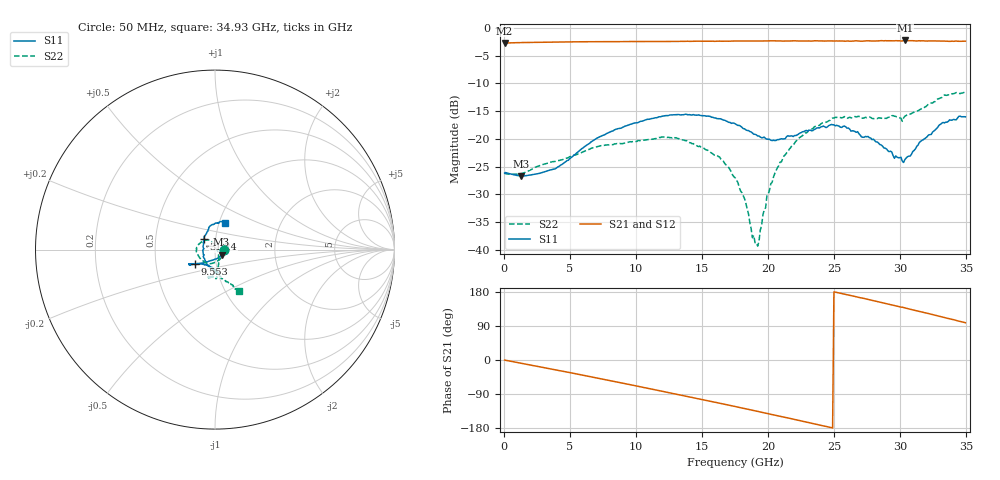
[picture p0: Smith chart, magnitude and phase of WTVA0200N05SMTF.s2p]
! 50 ohm 2-Port S-parameters measured by Modelithics Inc support@modelithics.com  Tampa, FL USA 813-866-6335 (February 2024)
! Smiths Interconnect,  2dB P/N: WTVA0200N05SMTF, Temperature: -25 C
! Board: 10 mil Rogers 4350B, Mounting Pad Dimensions: Length: 15 mils, Width: 25 mils, Gap: 40 mils.
# Hz S RI R 50
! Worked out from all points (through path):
!   352 points, 50 MHz to 34.93 GHz, reference 50 ohm
!   highest |S21| = -2.26 dB at 30.35 GHz (marker M1); lowest = -2.7 dB at 50 MHz (marker M2)
!   group delay of S21, straight-line fit = 20.8 ps
!   lowest |S11| = -26.7 dB at 1.294 GHz (marker M3), VSWR 1.10, Z = 53.7 - j3.05 ohm
!   |S11| at or under -10 dB: start of sweep to end of sweep
!   |S22| runs from -39.3 to -11.5 dB; largest |S21 - S12| = 0.0085
!   S11 on the Smith chart (normalised r, x): 50 MHz: 1.10, -0.00; 9.553 GHz: 0.79, -0.13; 31.24 GHz: 0.88, +0.11; 34.93 GHz: 1.07, +0.32
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5e7  0.0492 -0.00113  0.7303 -0.00271  0.7295 -0.00321  0.0499 -0.00106
1.2945e9  0.0368 -0.0283  0.7298 -0.1057  0.729 -0.1059  0.0395 -0.0285
3.8815e9  -0.00116 -0.0537  0.6713 -0.3221  0.6699 -0.3226  0.0212 -0.059
5.8715e9  -0.0441 -0.0684  0.5795 -0.4757  0.5784 -0.4758  -0.00984 -0.0747
9.553e9  -0.11 -0.0789  0.317 -0.684  0.3147 -0.684  -0.0752 -0.0572
1.1742e10  -0.1372 -0.0793  0.1212 -0.7442  0.1189 -0.7438  -0.1016 -0.0175
1.54235e10  -0.1364 -0.085  -0.2273 -0.7233  -0.2292 -0.7215  -0.0596 0.052
1.6319e10  -0.127 -0.0834  -0.3093 -0.6942  -0.3113 -0.6926  -0.041 0.0554
1.7513e10  -0.1096 -0.0812  -0.4133 -0.6396  -0.4149 -0.6375  -0.0164 0.0414
1.8309e10  -0.0912 -0.0791  -0.4769 -0.5927  -0.4778 -0.591  -0.000634 0.0264
1.88065e10  -0.081 -0.0791  -0.5161 -0.5601  -0.5169 -0.558  0.00537 0.0117
1.92045e10  -0.0689 -0.0807  -0.5441 -0.5329  -0.5453 -0.5306  0.0107 -0.00151
1.9901e10  -0.0526 -0.0846  -0.5911 -0.4824  -0.5913 -0.4808  0.0188 -0.0241
2.05975e10  -0.0326 -0.0913  -0.6351 -0.4239  -0.6363 -0.4207  0.0202 -0.0479
2.17915e10  -0.0123 -0.1059  -0.6928 -0.3192  -0.6929 -0.3169  0.0192 -0.0847
2.33835e10  0.00876 -0.1187  -0.7445 -0.1679  -0.7441 -0.1655  0.00257 -0.1241
2.57715e10  0.00637 -0.1304  -0.756 0.0848  -0.7549 0.0868  -0.0341 -0.1552
2.91545e10  -0.0575 -0.0508  -0.6427 0.4188  -0.6397 0.4216  0.0026 -0.1571
3.03485e10  -0.0647 0.00847  -0.5659 0.523  -0.5624 0.5253  0.0345 -0.1567
3.1244e10  -0.061 0.0601  -0.4901 0.5837  -0.4862 0.5859  0.0526 -0.1698
3.3234e10  -0.0146 0.1401  -0.2969 0.6994  -0.2924 0.7005  0.1157 -0.2132
3.49255e10  0.0572 0.1475  -0.1112 0.7514  -0.104 0.7514  0.133 -0.2304
